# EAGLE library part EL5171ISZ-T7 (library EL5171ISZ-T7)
Differential Amplifiers 250MHz Differential Twisted-Pair Drivers Source: Datasheet
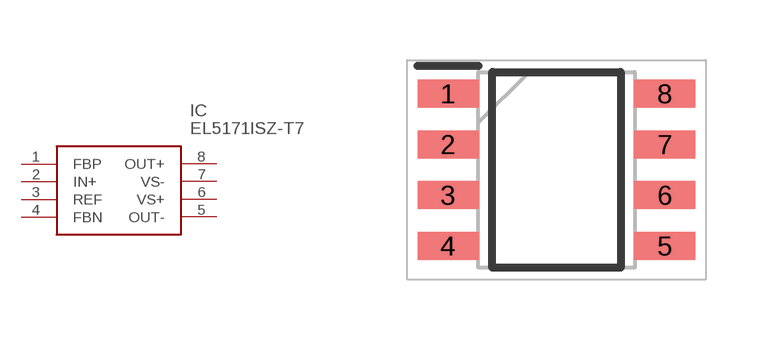
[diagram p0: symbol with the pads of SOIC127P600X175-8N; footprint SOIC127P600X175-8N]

Designator prefix IC

## EL5171ISZ-T7 (Description: Differential Amplifiers 250MHz Differential Twisted-Pair Drivers; Height: 1.75mm; Manufacturer_Name: Renesas Electronics; Manufacturer_Part_Number: EL5171ISZ-T7; Mouser_Part_Number: 968-EL5171ISZ-T7; Mouser_Price-Stock: https://www.mouser.co.uk/ProductDetail/Renesas-Intersil/EL5171ISZ-T7?qs=cbl4%252BYHJGOGN64pxrNVY0w%3D%3D)  [SOIC127P600X175-8N]
1  FBP
2  IN+
3  REF
4  FBN
5  OUT-
6  VS+
7  VS-
8  OUT+

## Footprint SOIC127P600X175-8N (pad centres in mm)
8 LEAD NARROW BODY SMALL OUTLINE PLASTIC PACKAGE
smd 1.525 x 0.7: 1 -2.712,1.905; 2 -2.712,0.635; 3 -2.712,-0.635; 4 -2.712,-1.905; 5 2.712,-1.905; 6 2.712,-0.635; 7 2.712,0.635; 8 2.712,1.905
